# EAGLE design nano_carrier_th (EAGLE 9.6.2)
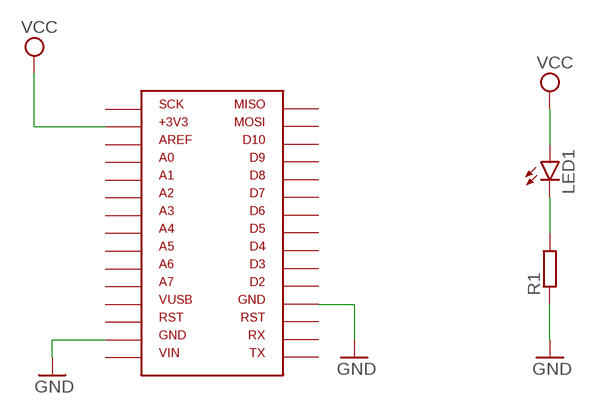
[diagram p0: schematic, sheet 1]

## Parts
LED1  LEDCHIPLED_0603  [CHIPLED_0603]
R1  SMK  [SMK]
U$1  NANO-TH  [NANO-TH]

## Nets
GND: R1.2 U$1.P$14 U$1.P$19
N$1: LED1.C R1.1
VCC: LED1.A U$1.P$2
Unconnected: U$1.P$1 U$1.P$3 U$1.P$4 U$1.P$5 U$1.P$6 U$1.P$7 U$1.P$8 U$1.P$9 U$1.P$10 U$1.P$11 U$1.P$12 U$1.P$13 U$1.P$15 U$1.P$16 U$1.P$17 U$1.P$18 U$1.P$20 U$1.P$21 U$1.P$22 U$1.P$23 U$1.P$24 U$1.P$25 U$1.P$26 U$1.P$27 U$1.P$28 U$1.P$29 U$1.P$30

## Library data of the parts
LED1 = led:LED: LED
R1 = resistor-shunt:SMK: SMD SHUNT RESISTOR; OC_FARNELL: unknown; OC_NEWARK: unknown
U$1 = Arduino-headers:NANO-TH

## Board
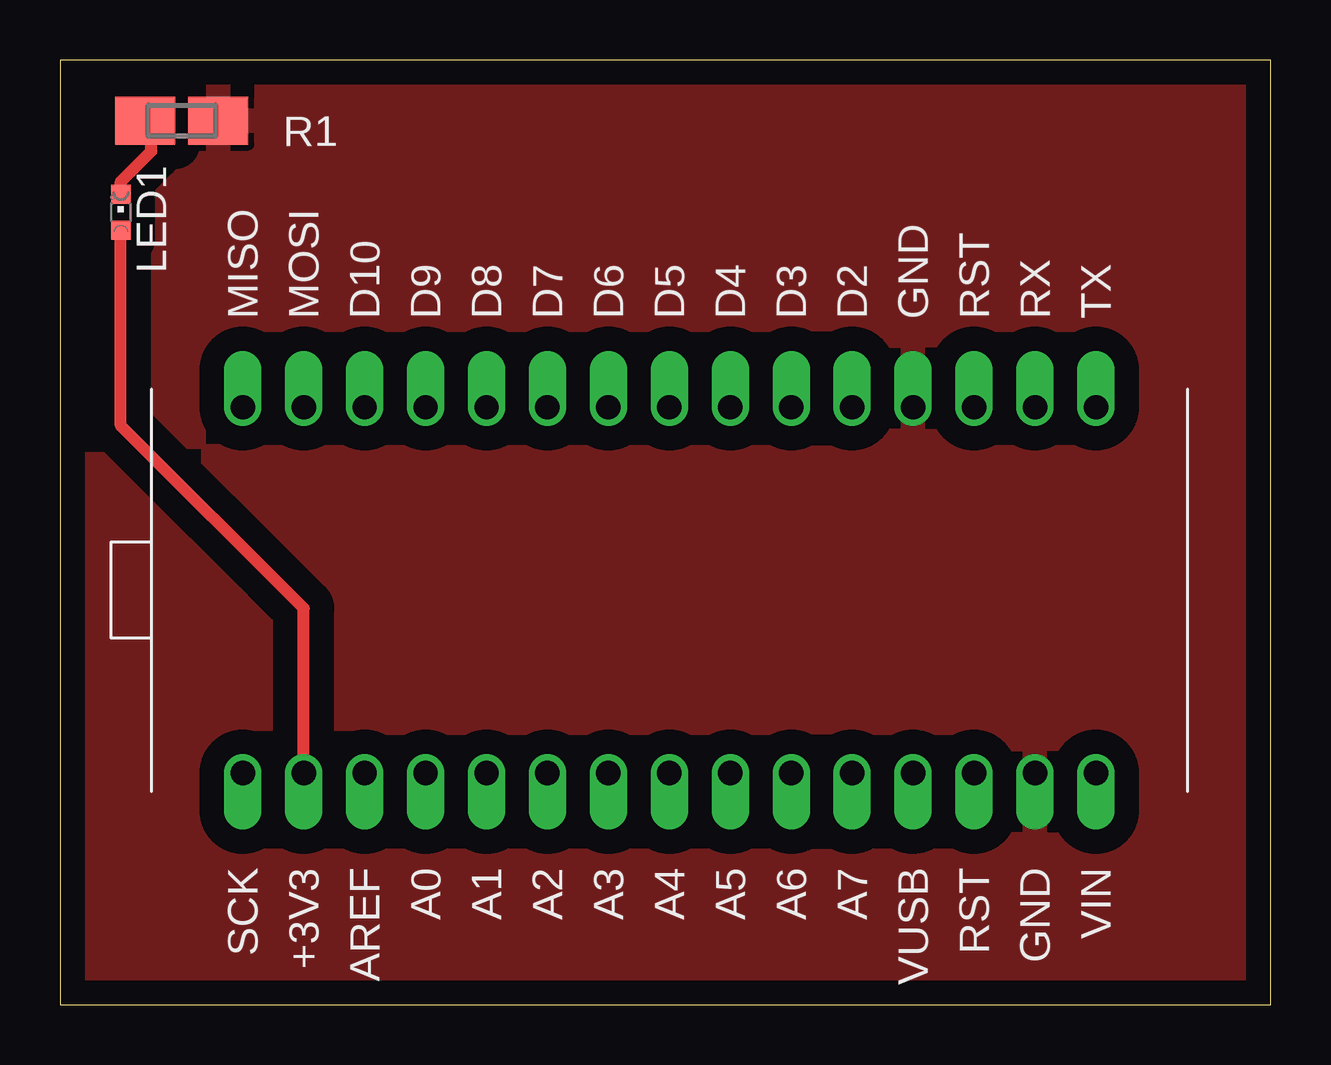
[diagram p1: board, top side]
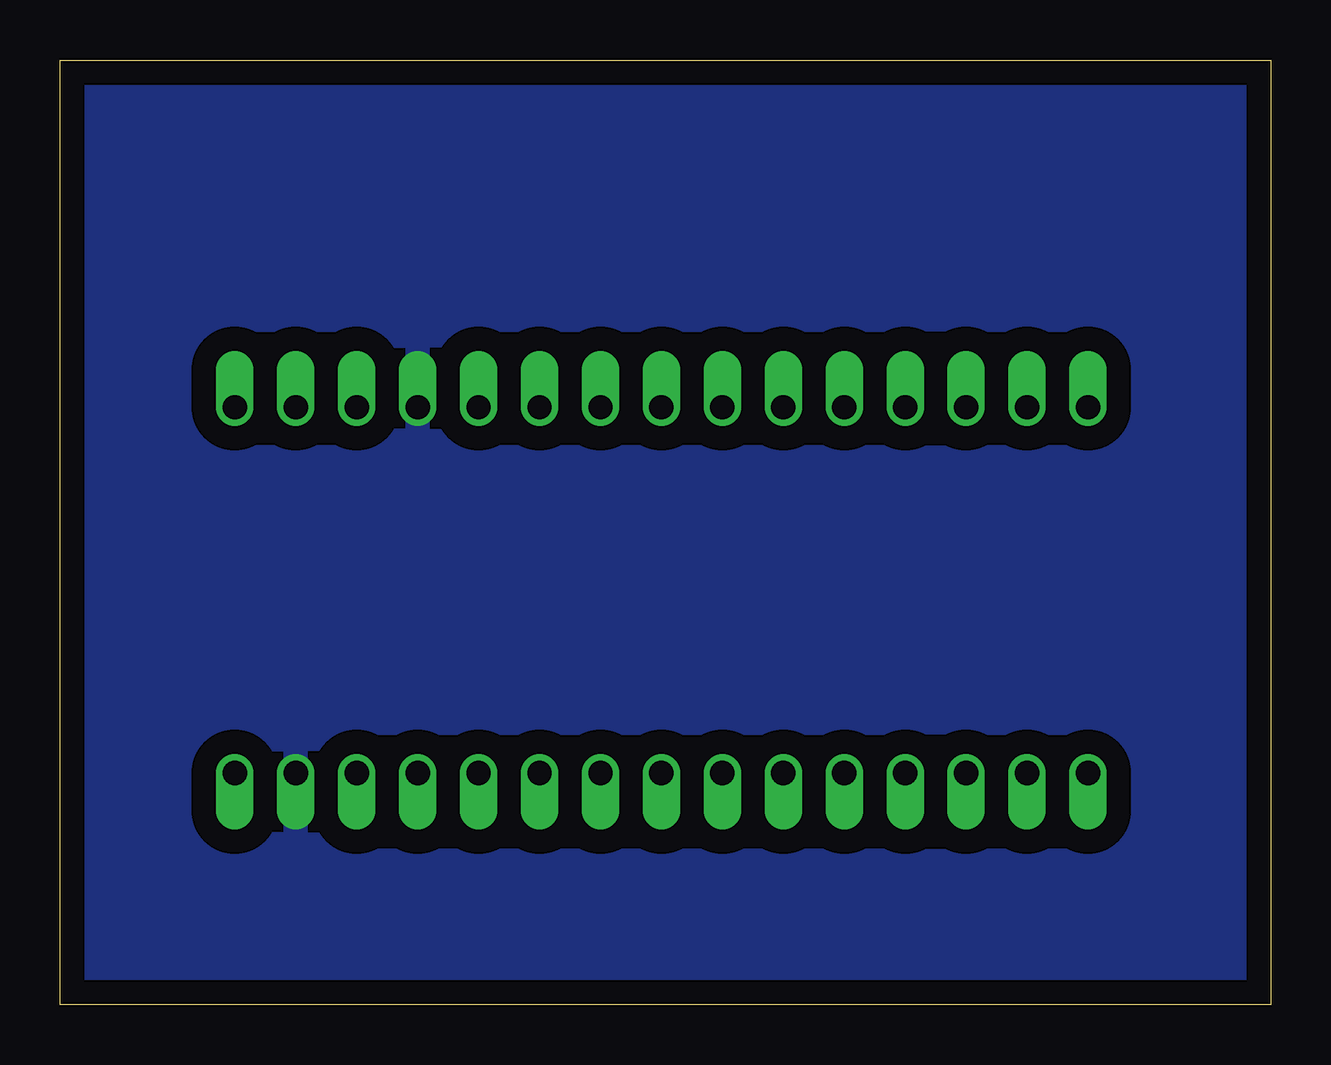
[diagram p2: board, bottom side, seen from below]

Size 50.47 x 39.36 mm. Coordinates in mm from the lower left corner, seen from the top.
Outline: 0,0 50.47,0 50.47,39.36 0,39.36 0,0
Copper layers (1*16): Top 0.035mm / dielectric 1.5mm / Bottom 0.035mm
Design rules "default": minimum track width 6mil, minimum drill 0.35mm, track to track 6mil, track to pad 6mil, pad to pad 6mil, via to via 6mil, smd to smd 6mil, copper to edge 40mil, drill to drill 6mil, minimum pad ring 10mil, minimum via ring 8mil, stop-mask expansion 4mil, vias tented up to drill 0mil, thermal gap 10mil

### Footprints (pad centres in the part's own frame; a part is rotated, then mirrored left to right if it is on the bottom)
CHIPLED_0603 = smd 0.8 x 0.8: A 0,-0.75; C 0,0.75
SMK = smd 2.5 x 2: 1 1.524,0; 2 -1.524,0
NANO-TH = drill 1.016 pad 1.57 offset: P$1 0,0.762; P$2 2.54,0.762; P$3 5.08,0.762; P$4 7.62,0.762; P$5 10.16,0.762; P$6 12.7,0.762; P$7 15.24,0.762; P$8 17.78,0.762; P$9 20.32,0.762; P$10 22.86,0.762; P$11 25.4,0.762; P$12 27.94,0.762; P$13 30.48,0.762; P$14 33.02,0.762; P$15 35.56,0.762; P$16 35.56,16.002; P$17 33.02,16.002; P$18 30.48,16.002; P$19 27.94,16.002; P$20 25.4,16.002; P$21 22.86,16.002; P$22 20.32,16.002; P$23 17.78,16.002; P$24 15.24,16.002; P$25 12.7,16.002; P$26 10.16,16.002; P$27 7.62,16.002; P$28 5.08,16.002; P$29 2.54,16.002; P$30 0,16

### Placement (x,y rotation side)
LED1  2.54,33.02 0 top
R1  5.08,36.83 180 top
U$1  7.62,8.89 0 top

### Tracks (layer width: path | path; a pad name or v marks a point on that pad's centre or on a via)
GND
  pour Top (isolate 1.016): 0,39.37 0,0 50.8,0 50.8,39.37
  pour Bottom (isolate 1.016): 0,39.37 0,0 50.8,0 50.8,39.37
N$1
  Top 0.508: LED1.C 2.54,34.29 3.81,35.56 3.81,36.58 R1.1
VCC
  Top 0.508: LED1.A 2.54,24.13 10.16,16.51 U$1.P$2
